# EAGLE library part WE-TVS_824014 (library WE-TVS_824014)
TVS Diode Array WE-TVS, Super Speed Serie - Low capazity - No leakage current - Low clamping voltage - high ESD voltage protection -- SATA -- DisplayPort -- DVI -- HDMI
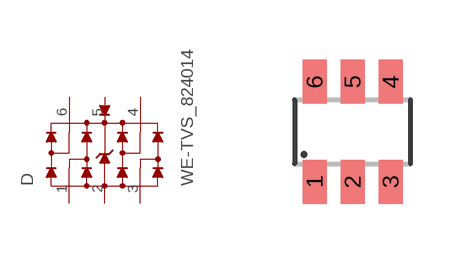
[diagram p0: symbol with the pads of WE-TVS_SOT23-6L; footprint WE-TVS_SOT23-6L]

Designator prefix D

## WE-TVS_824014 (MPN: 824014; OC_FARNELL: 1748614; OC_NEWARK: 34R6121; PACKAGE: SOT23-6L; SUPPLIER: Wuerth Elektronik)  [WE-TVS_SOT23-6L]
1  1  pas
2  GND  pwr
3  2  pas
4  3  pas
5  VDD  pwr
6  4  pas

## Footprint WE-TVS_SOT23-6L (pad centres in mm)
TVS Diode Array WE-TVS
smd 0.6 x 1.1: 1 -0.95,-1.25; 2 0,-1.25; 3 0.95,-1.25; 4 0.95,1.25; 5 0,1.25; 6 -0.95,1.25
